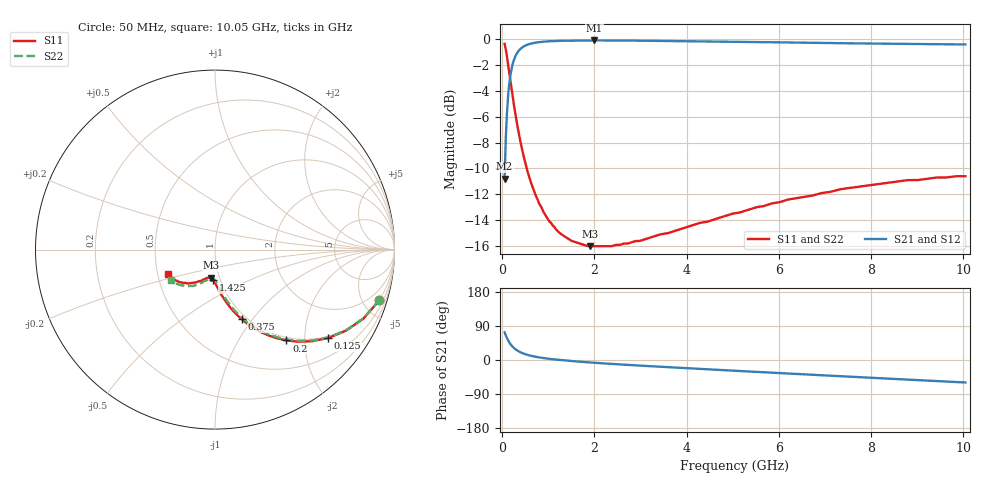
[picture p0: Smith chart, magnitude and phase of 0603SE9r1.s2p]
! AVX Thin Film Operation		Date: August 2001
! Description: Accu-P® Series, Thin Film, SMD, RF Capacitor
! Part Number: 06035J9R1BBT
! 50 MHz  -  10.05 GHz
! Serial Measurements
# mhz S db R 50
!	S11		S21		S12		S22
!	dB	Phase	dB	Phase	dB	Phase	dB	Phase
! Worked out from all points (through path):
!   401 points, 50 MHz to 10.05 GHz, reference 50 ohm
!   highest |S21| = -0.12 dB at 2 GHz (marker M1); lowest = -10.8 dB at 50 MHz (marker M2)
!   group delay of S21, straight-line fit = 21.1 ps
!   lowest |S11| = -16.0 dB at 1.9 GHz (marker M3), VSWR 1.38, Z = 45.6 - j14.7 ohm
!   |S11| at or under -10 dB: 530.6 MHz to end of sweep
!   |S22| runs from -16.0 to -0.4 dB; largest |S21 - S12| = 0
!   S11 on the Smith chart (normalised r, x): 50 MHz: 0.95, -6.48; 125 MHz: 0.95, -2.60; 200 MHz: 0.95, -1.64; 375 MHz: 0.95, -0.89; 1.425 GHz: 0.93, -0.32; 10.05 GHz: 0.57, -0.17
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50  -0.38 -17.2  -10.80 72.9  -10.80 72.9  -0.38 -17.0
75  -0.80 -25.0  -7.74 65.1  -7.74 65.1  -0.80 -24.7
125  -1.94 -38.0  -4.45 52.1  -4.45 52.1  -1.94 -37.7
150  -2.57 -43.3  -3.50 46.9  -3.50 46.9  -2.57 -42.9
200  -3.82 -51.8  -2.33 38.4  -2.33 38.4  -3.82 -51.2
275  -5.60 -61.0  -1.40 29.4  -1.40 29.4  -5.60 -60.2
375  -7.61 -68.9  -0.83 21.5  -0.83 21.5  -7.61 -67.9
450  -8.85 -73.1  -0.61 17.5  -0.61 17.5  -8.85 -71.8
550  -10.26 -77.3  -0.44 13.4  -0.44 13.4  -10.26 -75.7
675  -11.60 -81.1  -0.32 9.7  -0.32 9.7  -11.60 -79.3
825  -12.87 -84.6  -0.23 6.3  -0.23 6.3  -12.87 -82.4
1050  -14.18 -88.5  -0.17 2.6  -0.17 2.6  -14.18 -85.9
1425  -15.41 -93.3  -0.13 -2.0  -0.13 -2.0  -15.41 -90.2
1725  -15.85 -96.4  -0.12 -4.9  -0.12 -4.9  -15.85 -93.0
1900  -16.00 -98.0  -0.12 -6.5  -0.12 -6.5  -16.00 -94.3
2000  -16.00 -98.9  -0.12 -7.3  -0.12 -7.3  -16.00 -95.2
2725  -15.79 -105.0  -0.12 -12.9  -0.12 -12.9  -15.79 -101.0
3400  -15.12 -109.8  -0.14 -17.7  -0.14 -17.7  -15.12 -104.9
5050  -13.46 -120.4  -0.21 -28.5  -0.21 -28.5  -13.42 -115.4
6725  -12.10 -132.0  -0.30 -38.9  -0.30 -38.9  -12.00 -126.0
8400  -11.09 -142.2  -0.37 -49.3  -0.37 -49.3  -11.09 -135.2
10050  -10.60 -152.8  -0.42 -59.4  -0.42 -59.4  -10.52 -144.8
